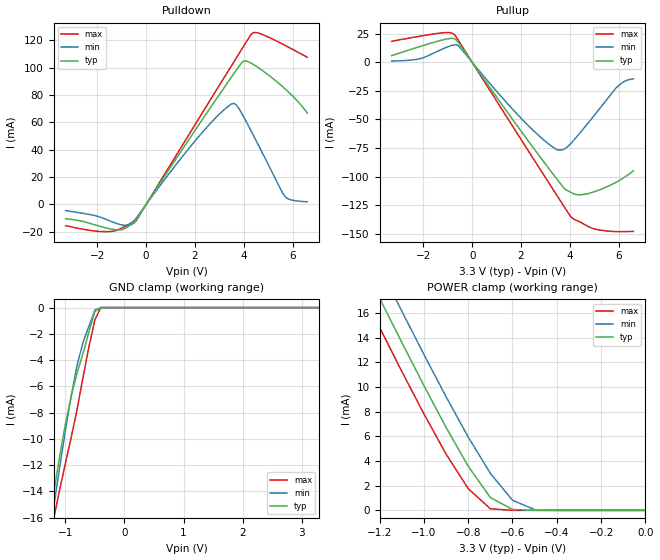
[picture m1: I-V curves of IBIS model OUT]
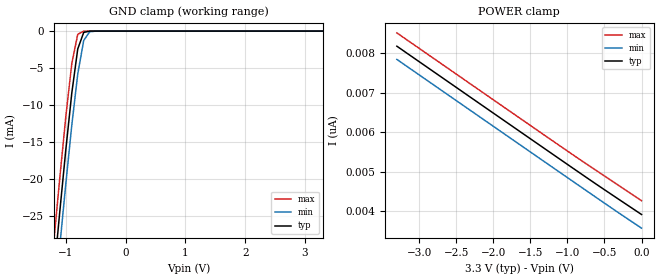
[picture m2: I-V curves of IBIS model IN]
|   TEXAS INSTRUMENTS INCORPORATED
|   Standard Linear and Logic
|   IBIS Model of SN74ALVC162334
|   16-BIT Universal Bus Driver with 3-state outputs
|   48-pin DGG, DGV, or DL Package
[IBIS Ver]   2.1
[Comment char]  |_char
[File Name]   alvc162334.ibs
[File Rev]   2.0
[Date]   9/29/98
[Source]   File originated at Texas Instruments, Inc.
[Notes]   The following is an IBIS list for the ALVC162334.
|   - This file may be incomplete or may not be fully compliant
|   with the IBIS specification. It will be replaced with a
|   version that is IBIS Revision 3.2 compliant and is complete
|   and accurate.  Please email all questions and comments to
|   sllibis@ti.com.
|   - All test data contained in this file are derived from
|   hspice(tm) simulations.
|   - File created by David Yaeger, SLL Applications
[Disclaimer]
* Property of Texas Instruments Incorporated.  Unauthorized *
* reproduction and/or distribution is strictly prohibited. *
* This product is protected under copyright law. *
* Created 1997, (C) Copyright 1997, Texas Instruments Inc., *
* All Rights Reserved *
* UNLESS THERE IS A SIGNED, WRITTEN AGREEMENT TO THE *
* CONTRARY, TEXAS INSTRUMENTS ("TI") IS PROVIDING THE IBIS *
* MODELS "AS IS" AND WITHOUT ANY WARRANTY, EXPRESSED OR *
* IMPLIED.  TI assumes no liability for: *
* 1) the accuracy of the IBIS models provided to your *
* company; *
* 2) the proper functioning of these IBIS models in your *
* design or for any resulting applications; or *
* 3) infringement of patents, copyrights or intellectual *
* property rights resulting from your use of these *
* IBIS models. *
* TI provides IBIS Models as a service to our customers. *
* You and your company shall not distribute, sell or give *
* these models to anyone else without prior written *
* permission from TI. *
* TI reserves the right to make changes to our products or *
* to discontinue any semiconductor product or service *
* without notice, and advises our customers to obtain the *
* latest version of relevant information to verify, before *
* placing orders, that the information being relied on is *
* current. *
* Please be aware that your receipt and use of the IBIS *
* information provided shall serve as acceptance of these *
* terms and conditions.  If you do not accept these terms, *
* you should return or destroy the IBIS models and any *
* other accompanying information immediately. *
[Component]   ALVC162334_DGG
[Manufacturer]  Texas Instruments, Inc.
[Package]
|   typ   min   max
R_pkg   0.056   0.039   0.068
L_pkg   3.39nH   3.078nH   3.995nH
C_pkg   0.52pF   0.414pF   0.668pF
[Pin]   signal_name   model_name   R_pin   L_pin   C_pin
1   OE_BAR   NC   0.039   3.987nH   0.654pF
2   Y1   OUT   0.047   3.725nH   0.659pF
3   Y2   OUT   0.059   3.692nH   0.604pF
4   GND   GND   0.068   3.675nH   0.606pF
5   Y3   OUT   0.055   3.473nH   0.547pF
6   Y4   OUT   0.056   3.402nH   0.497pF
7   VCC   POWER   0.057   3.3nH   0.492pF
8   Y5   OUT   0.056   3.189nH   0.455pF
9   Y6   OUT   0.058   3.154nH   0.449pF
10   GND   GND   0.058   3.094nH   0.436pF
11   Y7   OUT   0.058   3.078nH   0.424pF
12   Y8   OUT   0.06   3.081nH   0.414pF
13   Y9   OUT   0.061   3.097nH   0.416pF
14   Y10   OUT   0.06   3.126nH   0.427pF
15   GND   GND   0.061   3.158nH   0.44pF
16   Y11   OUT   0.058   3.173nH   0.45pF
17   Y12   OUT   0.056   3.189nH   0.455pF
18   VCC   POWER   0.056   3.265nH   0.49pF
19   Y13   OUT   0.054   3.322nH   0.492pF
20   Y14   OUT   0.052   3.388nH   0.544pF
21   GND   GND   0.064   3.591nH   0.605pF
22   Y15   OUT   0.059   3.677nH   0.612pF
23   Y16   OUT   0.046   3.678nH   0.668pF
24   NC   NC   0.041   3.979nH   0.659pF
25   LE_BAR   NC   0.04   3.995nH   0.658pF
26   A16   IN   0.046   3.69nH   0.662pF
27   A15   IN   0.057   3.649nH   0.602pF
28   GND   GND   0.066   3.615nH   0.602pF
29   A14   IN   0.055   3.447nH   0.547pF
30   A13   IN   0.054   3.326nH   0.492pF
31   VCC   POWER   0.055   3.239nH   0.488pF
32   A12   IN   0.056   3.183nH   0.454pF
33   A11   IN   0.057   3.144nH   0.447pF
34   GND   GND   0.058   3.099nH   0.436pF
35   A10   IN   0.059   3.086nH   0.425pF
36   A9   IN   0.06   3.081nH   0.414pF
37   A8   IN   0.061   3.097nH   0.415pF
38   A7   IN   0.06   3.119nH   0.427pF
39   GND   GND   0.06   3.144nH   0.439pF
40   A6   IN   0.056   3.13nH   0.446pF
41   A5   IN   0.057   3.208nH   0.456pF
42   VCC   POWER   0.056   3.247nH   0.487pF
43   A4   IN   0.054   3.328nH   0.491pF
44   A3   IN   0.053   3.413nH   0.546pF
45   GND   GND   0.066   3.609nH   0.606pF
46   A2   IN   0.058   3.689nH   0.607pF
47   A1   IN   0.047   3.727nH   0.662pF
48   CLK   NC   0.04   3.978nH   0.655pF
[Component]   ALVC162334_DGV
[Manufacturer]  Texas Instruments, Inc.
[Package]
|   typ   min   max
R_pkg   0.063   0.043   0.09
L_pkg   3.077nH   2.377nH   4.305nH
C_pkg   0.387pF   0.281pF   0.565pF
[Pin]   signal_name   model_name   R_pin   L_pin   C_pin
1   OE_BAR   NC   0.082   4.277nH   0.562pF
2   Y1   OUT   0.09   4.02nH   0.554pF
3   Y2   OUT   0.087   3.719nH   0.478pF
4   GND   GND   0.087   3.456nH   0.417pF
5   Y3   OUT   0.076   3.207nH   0.411pF
6   Y4   OUT   0.044   2.929nH   0.39pF
7   VCC   POWER   0.046   2.803nH   0.335pF
8   Y5   OUT   0.047   2.683nH   0.321pF
9   Y6   OUT   0.048   2.579nH   0.311pF
10   GND   GND   0.049   2.505nH   0.302pF
11   Y7   OUT   0.048   2.4nH   0.289pF
12   Y8   OUT   0.051   2.4nH   0.283pF
13   Y9   OUT   0.051   2.4nH   0.283pF
14   Y10   OUT   0.05   2.433nH   0.291pF
15   GND   GND   0.048   2.46nH   0.298pF
16   Y11   OUT   0.048   2.585nH   0.312pF
17   Y12   OUT   0.046   2.652nH   0.319pF
18   VCC   POWER   0.045   2.787nH   0.336pF
19   Y13   OUT   0.046   2.962nH   0.394pF
20   Y14   OUT   0.074   3.208nH   0.409pF
21   GND   GND   0.087   3.488nH   0.417pF
22   Y15   OUT   0.087   3.741nH   0.478pF
23   Y16   OUT   0.089   3.99nH   0.546pF
24   NC   NC   0.084   4.305nH   0.557pF
25   LE_BAR   NC   0.082   4.286nH   0.565pF
26   A16   IN   0.086   3.933nH   0.554pF
27   A15   IN   0.086   3.699nH   0.475pF
28   GND   GND   0.089   3.522nH   0.42pF
29   A14   IN   0.079   3.234nH   0.413pF
30   A13   IN   0.043   2.88nH   0.385pF
31   VCC   POWER   0.045   2.779nH   0.332pF
32   A12   IN   0.045   2.636nH   0.317pF
33   A11   IN   0.047   2.553nH   0.309pF
34   GND   GND   0.048   2.468nH   0.298pF
35   A10   IN   0.05   2.424nH   0.29pF
36   A9   IN   0.05   2.377nH   0.281pF
37   A8   IN   0.05   2.387nH   0.281pF
38   A7   IN   0.05   2.431nH   0.29pF
39   GND   GND   0.048   2.475nH   0.299pF
40   A6   IN   0.048   2.557nH   0.309pF
41   A5   IN   0.047   2.671nH   0.319pF
42   VCC   POWER   0.046   2.804nH   0.334pF
43   A4   IN   0.044   2.935nH   0.39pF
44   A3   IN   0.074   3.203nH   0.412pF
45   GND   GND   0.085   3.444nH   0.416pF
46   A2   IN   0.085   3.723nH   0.477pF
47   A1   IN   0.09   4.012nH   0.547pF
48   CLK   NC   0.083   4.288nH   0.558pF
[Component]   ALVC162334_DL
[Manufacturer]  Texas Instruments, Inc.
[Package]
|   typ   min   max
R_pkg   0.048   0.038   0.053
L_pkg   6.046nH   5.084nH   7.968nH
C_pkg   0.813pF   0.569pF   1.157pF
[Pin]   signal_name   model_name   R_pin   L_pin   C_pin
1   OE_BAR   NC   0.046   7.968nH   1.017pF
2   Y1   OUT   0.044   7.299nH   1.157pF
3   Y2   OUT   0.043   6.765nH   1.058pF
4   GND   GND   0.041   6.269nH   0.933pF
5   Y3   OUT   0.038   5.856nH   0.829pF
6   Y4   OUT   0.046   5.802nH   0.79pF
7   VCC   POWER   0.05   5.656nH   0.738pF
8   Y5   OUT   0.053   5.5nH   0.643pF
9   Y6   OUT   0.052   5.304nH   0.606pF
10   GND   GND   0.053   5.189nH   0.583pF
11   Y7   OUT   0.051   5.084nH   0.569pF
12   Y8   OUT   0.053   5.862nH   0.833pF
13   Y9   OUT   0.053   5.862nH   0.833pF
14   Y10   OUT   0.051   5.084nH   0.569pF
15   GND   GND   0.053   5.189nH   0.583pF
16   Y11   OUT   0.052   5.304nH   0.606pF
17   Y12   OUT   0.053   5.5nH   0.643pF
18   VCC   POWER   0.05   5.656nH   0.738pF
19   Y13   OUT   0.046   5.802nH   0.79pF
20   Y14   OUT   0.038   5.856nH   0.829pF
21   GND   GND   0.041   6.269nH   0.933pF
22   Y15   OUT   0.043   6.765nH   1.058pF
23   Y16   OUT   0.044   7.299nH   1.157pF
24   NC   NC   0.046   7.968nH   1.017pF
25   LE_BAR   NC   0.046   7.968nH   1.017pF
26   A16   IN   0.044   7.299nH   1.157pF
27   A15   IN   0.043   6.765nH   1.058pF
28   GND   GND   0.041   6.269nH   0.933pF
29   A14   IN   0.038   5.856nH   0.829pF
30   A13   IN   0.046   5.802nH   0.79pF
31   VCC   POWER   0.05   5.656nH   0.738pF
32   A12   IN   0.053   5.5nH   0.643pF
33   A11   IN   0.052   5.304nH   0.606pF
34   GND   GND   0.053   5.189nH   0.583pF
35   A10   IN   0.051   5.084nH   0.569pF
36   A9   IN   0.053   5.862nH   0.833pF
37   A8   IN   0.053   5.862nH   0.833pF
38   A7   IN   0.051   5.084nH   0.569pF
39   GND   GND   0.053   5.189nH   0.583pF
40   A6   IN   0.052   5.304nH   0.606pF
41   A5   IN   0.053   5.5nH   0.643pF
42   VCC   POWER   0.05   5.656nH   0.738pF
43   A4   IN   0.046   5.802nH   0.79pF
44   A3   IN   0.038   5.856nH   0.829pF
45   GND   GND   0.041   6.269nH   0.933pF
46   A2   IN   0.043   6.765nH   1.058pF
47   A1   IN   0.044   7.299nH   1.157pF
48   CLK   NC   0.046   7.967nH   1.017pF
| Models and submodels in the file (2): OUT (3-state), IN (Input)
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|   Model ALVC162334_OUT
[Model]   OUT
Model_type   3-state
Polarity   Non-Inverting
Enable   Active-High
|Variable   typ   min   max
C_comp   7.0pF   NA   NA
[Voltage range]   3.3   3.0   3.6
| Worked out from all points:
|   slope of the pulldown table from 0 to 0.495 V, typ, clamps not added: 36.6 ohm
|   slope of the pullup table from 0 to 0.495 V, typ, clamps not added: 32.7 ohm
|   GND clamp passes 1 mA (typ) near -0.55 V on its own axis
|   POWER clamp passes 1 mA (typ) near -0.70 V on its own axis
[Pullup]   | Note: Vtable = Vcc - Voutput
|   Voltage   I(typ)   I(min)   I(max)
-3.3V     5.885mA    1.117mA    18.39mA
-2.1V     14.11mA    3.456mA    23.04mA
-1V       20.6mA     13.61mA    26.08mA
-700mV    20.46mA    15.34mA    23.61mA
2.1V      -63.06mA   -51.09mA   -70.81mA
3.5V      -103mA     -76.72mA   -117.5mA
3.8V      -111mA     -75.68mA   -127.4mA
4.1V      -114.5mA   -69.58mA   -136.4mA
4.5V      -115.8mA   -59.55mA   -140.6mA
5V        -113.2mA   -46.36mA   -145.7mA
5.9V      -104.9mA   -22.26mA   -148.1mA
6.6V      -94.9mA    -14.44mA   -147.9mA
[Pulldown]
|   Voltage   I(typ)   I(min)   I(max)
-3.3V     -10.48mA   -4.527mA   -15.6mA
-2V       -15.48mA   -8.665mA   -19.65mA
-1.2V     -18.63mA   -14.02mA   -18.88mA
-800mV    -16.93mA   -15.16mA   -15.62mA
-500mV    -13.4mA    -12.01mA   -13.67mA
2.2V      59.34mA    50.53mA    63.98mA
3.1V      82.92mA    67.69mA    89.97mA
3.6V      95.76mA    73.79mA    104.4mA
4V        104.8mA    63.73mA    115.8mA
4.4V      102.1mA    50.15mA    125.5mA
5.7V      84.22mA    5.448mA    116.1mA
6.6V      66.66mA    1.873mA    107.4mA
[POWER_Clamp]   | Note: Vtable = Vcc - Voutput
|   Voltage   I(typ)   I(min)   I(max)
-3.3V     95.82mA    98.2mA     93.52mA
-1.3V     20.85mA    23.37mA    18.46mA
-1.2V     17.22mA    19.76mA    14.85mA
-1.1V     13.64mA    16.18mA    11.29mA
-1V       10.13mA    12.66mA    7.835mA
-900mV    6.739mA    9.228mA    4.573mA
-800mV    3.582mA    5.956mA    1.766mA
-700mV    1.041mA    3.004mA    129uA
-600mV    70.56uA    819.7uA    1.512uA
-500mV    2.077uA    58.75uA    22.94nA
0V        990pA      903.2pA    1.08nA
[GND_Clamp]
|   Voltage   I(typ)   I(min)   I(max)
-3.3V     -82.07mA   -83.71mA   -80.7mA
-1.3V     -17.13mA   -18.37mA   -18.52mA
-1.2V     -14.21mA   -15.29mA   -16.14mA
-1.1V     -11.45mA   -12.28mA   -13.96mA
-1V       -8.904mA   -9.398mA   -11.89mA
-900mV    -6.72mA    -6.711mA   -9.882mA
-800mV    -4.963mA   -4.374mA   -7.729mA
-700mV    -3.48mA    -2.629mA   -5.291mA
-600mV    -1.837mA   -1.41mA    -2.981mA
-500mV    -287uA     -193.3uA   -927.2uA
-400mV    -9.992nA   -367.2nA   -984.6pA
3.3V      990pA      123.6nA    930pA
[Ramp]
| variable   typ   min   max
dV/dt_r   1.1975E+00/1.8907E-10  1.0066E+00/2.8668E-10  1.3583E+00/1.7118E-10
dV/dt_f   1.1452E+00/2.0047E-10  9.8613E-01/4.1927E-10  1.2876E+00/1.6417E-10
|   Model ALVC162334_IN
[Model]   IN
Model_type   Input
Polarity   Non-Inverting
Vinl = 0.8V
Vinh = 2.0V
|Variable   typ   min   max
C_comp   6pF   NA   NA
[Voltage Range]   3.3   3.0   3.6
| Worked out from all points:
|   GND clamp passes 1 mA (typ) near -0.74 V on its own axis
[POWER_Clamp]   | Note: Vtable = Vcc - Voutput
|   Voltage   I(typ)   I(min)   I(max)
-3.3V     8.169nA    7.835nA    8.505nA
-1V       5.186nA    4.852nA    5.523nA
-600mV    4.672nA    4.336nA    5.018nA
0V        3.921nA    3.575nA    4.268nA
[GND_Clamp]
|   Voltage   I(typ)   I(min)   I(max)
-3.3V     -226.9mA   -231.1mA   -222.8mA
-1.2V     -33.05mA   -37.73mA   -28.48mA
-1.1V     -24.41mA   -29.09mA   -19.85mA
-1V       -16.09mA   -20.7mA    -11.63mA
-900mV    -8.415mA   -12.77mA   -4.423mA
-800mV    -2.415mA   -5.819mA   -431.6uA
-700mV    -180.1uA   -1.262mA   -9.285uA
-600mV    -6.422uA   -95.7uA    -168.7nA
-500mV    -216.5nA   -5.198uA   -3.949nA
3.3V      3.921nA    3.952nA    3.894nA
